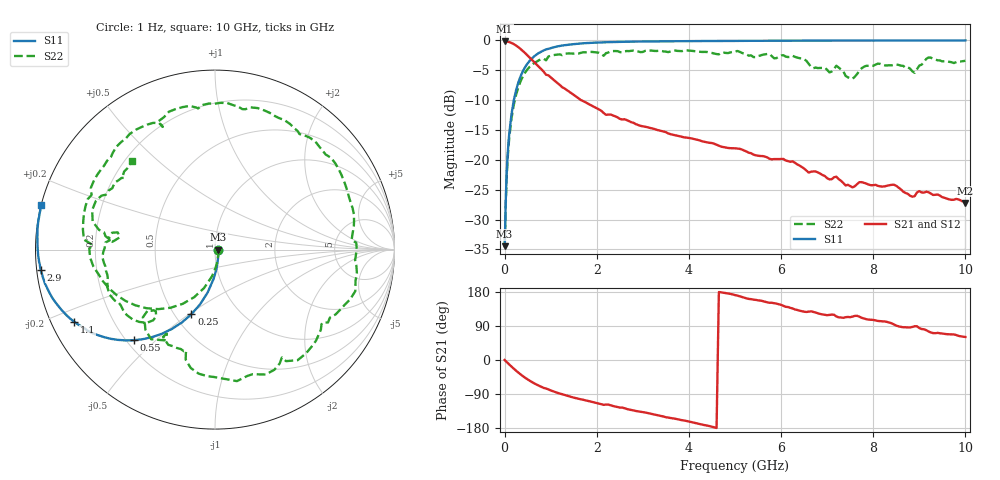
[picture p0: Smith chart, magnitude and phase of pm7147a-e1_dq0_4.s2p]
# GHz S DB R 50
! S-Parameters data
! Freq  dbS11  angS11  dbS21  angS21  dbS12  angS12  dbS22  angS22
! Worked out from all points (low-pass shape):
!   279 points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, 1 Hz to 10 GHz, reference 50 ohm
!   highest |S21| = -0.17 dB at 3.981 kHz (marker M1); lowest = -27.2 dB at 10 GHz (marker M2)
!   |S21| within 3 dB of the highest: start of sweep to 581.7 MHz
!   lowest |S11| = -34.5 dB at 3.162 kHz (marker M3), VSWR 1.04, Z = 51.9 - j0.000536 ohm
!   |S11| at or under -10 dB: start of sweep to 201 MHz
!   |S22| runs from -34.5 to -1.7 dB; largest |S21 - S12| = 2.1e-13
!   S11 on the Smith chart (normalised r, x): 1 Hz: 1.04, -0.00; 250 MHz: 0.60, -0.51; 550 MHz: 0.23, -0.43; 1.1 GHz: 0.07, -0.24; 2.9 GHz: 0.01, -0.06; 10 GHz: 0.00, +0.13
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1e-09  -34.47 -0.0  -0.17 -0.0  -0.17 -0.0  -34.47 -0.0
3.1623e-06  -34.47 -0.0  -0.17 -0.0  -0.17 -0.0  -34.47 -0.0
3.9811e-06  -34.47 -0.0  -0.17 -0.0  -0.17 -0.0  -34.47 -0.0
0.03981072  -23.31 -77.5  -0.19 -4.7  -0.19 -4.7  -23.96 -78.0
0.07943282  -17.62 -89.4  -0.24 -9.3  -0.24 -9.3  -18.30 -92.2
0.25  -8.33 -110.0  -0.87 -28.3  -0.87 -28.3  -9.09 -120.7
0.55  -3.36 -131.9  -2.92 -55.1  -2.92 -55.1  -4.38 -155.1
1.1  -1.10 -152.9  -6.86 -84.7  -6.86 -84.7  -2.42 164.7
1.7  -0.49 -163.4  -10.15 -104.8  -10.15 -104.8  -2.01 133.7
2.9  -0.19 -173.5  -14.18 -135.5  -14.18 -135.5  -1.87 80.6
3.35  -0.16 -175.8  -15.07 -146.5  -15.07 -146.5  -1.74 61.7
4.1  -0.12 -178.9  -16.50 -165.3  -16.50 -165.3  -1.79 28.0
5.05  -0.09 177.9  -18.12 170.0  -18.12 170.0  -1.77 -16.5
6.05  -0.06 175.0  -19.86 143.1  -19.86 143.1  -2.48 -67.9
6.7  -0.04 173.3  -21.95 126.9  -21.95 126.9  -4.66 -105.9
7.2  -0.04 172.1  -22.84 115.0  -22.84 115.0  -4.25 -125.5
7.4  -0.03 171.6  -24.29 113.0  -24.29 113.0  -5.94 -137.9
7.75  -0.03 170.7  -23.74 111.3  -23.74 111.3  -4.66 -136.5
8.35  -0.03 169.3  -24.27 98.8  -24.27 98.8  -4.17 -169.1
8.9  -0.02 168.1  -26.08 89.1  -26.08 89.1  -5.43 172.7
9.2  -0.02 167.5  -25.43 75.3  -25.43 75.3  -2.87 162.1
10  -0.01 165.7  -27.22 60.8  -27.22 60.8  -3.42 133.2
